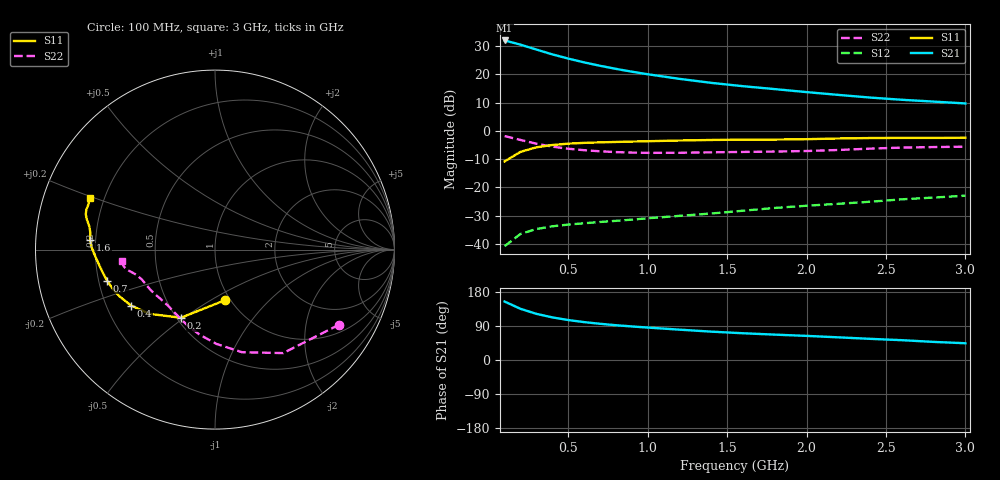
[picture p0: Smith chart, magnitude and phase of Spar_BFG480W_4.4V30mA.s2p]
! Filename: 4_430BFG480.001
! Title: BFG480W
! Bias: Vce=4.4V; Ic=30mA
! Company: NXP Semiconductors NL
! User: Quality&Reliability T&D
! Measure time: 10 Nov 1999 / 12:05:38
#  MHz  S  MA  R 50
! Freq  S11  S21  S12  S22  :
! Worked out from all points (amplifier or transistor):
!   20 points, 100 MHz to 3 GHz, reference 50 ohm
!   highest |S21| = 32.0 dB at 100 MHz (marker M1)
!   |S21| within 3 dB of that: start of sweep to 287.2 MHz
!   unconditionally stable (mu >= 1): 1.156 GHz to end of sweep
!   at 400 MHz: K = 0.52, MSG = 30.4 dB, |S12| = -33.8 dB
!   at 1.2 GHz: K = 1.02, MAG = 23.5 dB, |S12| = -30.1 dB
!   at 3 GHz: K = 1.07, MAG = 14.7 dB, |S12| = -23.0 dB
!   S11 on the Smith chart (normalised r, x): 100 MHz: 0.94, -0.58; 200 MHz: 0.53, -0.49; 400 MHz: 0.30, -0.28; 700 MHz: 0.23, -0.13; 1.6 GHz: 0.18, +0.04; 3 GHz: 0.15, +0.19
100  0.2878 -79.2  39.82 154.3  0.009089 60.7  0.8079 -31.2
200  0.4247 -116.6  33.56 135.1  0.01498 52.9  0.6904 -56.6
300  0.5115 -135.6  27.48 121.8  0.01827 47.6  0.5912 -75.2
400  0.5619 -146.3  22.59 112.5  0.02042 45.5  0.5254 -89.2
500  0.5933 -154.1  19.04 105.5  0.02189 45.1  0.4826 -99.9
600  0.6125 -159.7  16.3 100.0  0.02312 45.7  0.4543 -108.3
700  0.6256 -164.0  14.2 95.6  0.02434 47.2  0.4347 -115.0
800  0.6358 -167.6  12.52 91.8  0.02552 49.0  0.4209 -120.6
900  0.6455 -170.8  11.15 88.6  0.0268 51.3  0.4123 -125.6
1000  0.6554 -173.6  10.05 85.6  0.02832 53.3  0.4077 -130.1
1200  0.6744 -178.2  8.331 80.1  0.03127 56.9  0.4091 -137.7
1400  0.6896 178.4  7.076 74.8  0.03441 60.1  0.4168 -143.6
1600  0.6982 175.4  6.171 70.6  0.03854 63.1  0.4234 -148.0
1800  0.7008 172.3  5.481 67.0  0.04318 65.6  0.43 -152.4
2000  0.7118 169.6  4.851 63.6  0.04724 68.0  0.4392 -157.4
2200  0.7325 166.9  4.332 59.8  0.05109 69.1  0.4584 -162.0
2400  0.7463 164.7  3.884 55.8  0.05564 69.8  0.4842 -165.2
2600  0.7505 162.9  3.549 52.3  0.06132 70.2  0.5054 -167.3
2800  0.749 160.5  3.294 47.8  0.06596 69.6  0.5164 -169.5
3000  0.7546 157.6  3.057 44.2  0.07116 69.6  0.5248 -172.8
